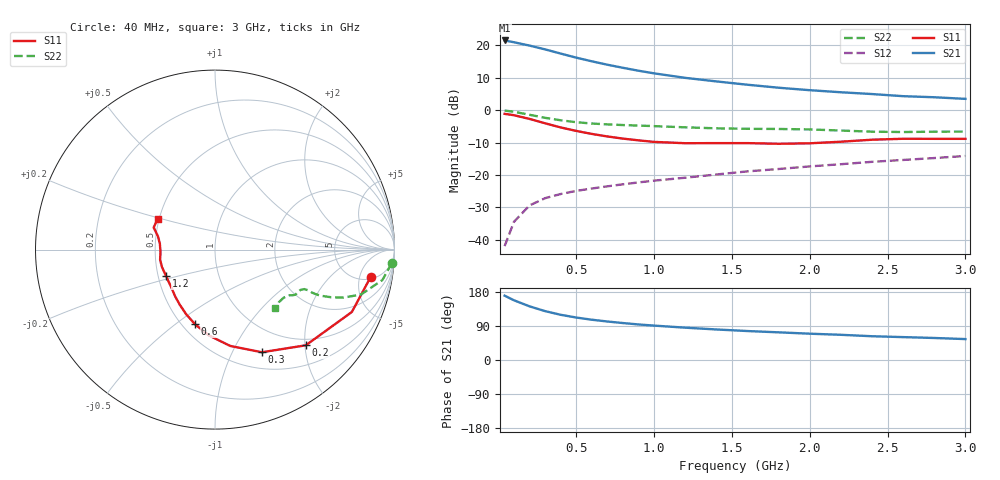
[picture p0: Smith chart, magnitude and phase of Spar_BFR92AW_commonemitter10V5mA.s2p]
! Filename:  BFR92AWG.S2P  Version:  4.0
! NXP part #: BFR92AW  Date: Jun 1994
! Bias condition: Vce=10V, Ic=5mA
#  MHz  S  MA  R  50
! Freq  S11  S21  S12  S22  !GUM [dB]
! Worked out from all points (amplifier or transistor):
!   21 points, 40 MHz to 3 GHz, reference 50 ohm
!   highest |S21| = 21.5 dB at 40 MHz (marker M1)
!   |S21| within 3 dB of that: start of sweep to 319.1 MHz
!   unconditionally stable (mu >= 1): 962.7 MHz to end of sweep
!   at 300 MHz: K = 0.48, MSG = 23.0 dB, |S12| = -27.1 dB
!   at 1 GHz: K = 1.02, MAG = 15.7 dB, |S12| = -21.7 dB
!   at 3 GHz: K = 1.14, MAG = 6.5 dB, |S12| = -14.1 dB
!   lowest NFmin = 1.60 dB at 500 MHz
!   S11 on the Smith chart (normalised r, x): 40 MHz: 5.41, -7.41; 200 MHz: 0.87, -2.02; 300 MHz: 0.69, -1.31; 600 MHz: 0.58, -0.59; 1.2 GHz: 0.55, -0.18; 3 GHz: 0.49, +0.19
40  0.88 -10.1  11.93 169.8  0.008 84.3  0.988 -4.4
100  0.838 -24.5  11.19 157.6  0.019 75.3  0.948 -10.3
200  0.735 -46.5  9.939 141.6  0.034 65.5  0.851 -17.1
300  0.629 -65.4  8.686 129.0  0.044 59.8  0.764 -20.5
400  0.543 -81.1  7.485 119.3  0.051 57.2  0.7 -22.3
500  0.48 -93.9  6.476 112.1  0.057 56.4  0.654 -23.3
600  0.431 -104.9  5.687 106.3  0.062 57.1  0.624 -23.8
700  0.394 -114.1  5.039 101.6  0.067 58.2  0.605 -23.9
800  0.365 -122.4  4.515 97.5  0.072 59.3  0.591 -23.9
900  0.343 -130.2  4.07 93.8  0.077 60.4  0.58 -23.7
1000  0.325 -137.5  3.708 90.8  0.082 61.6  0.569 -23.6
1200  0.31 -151.4  3.159 85.3  0.091 63.8  0.545 -23.8
1400  0.311 -161.9  2.785 80.6  0.102 66.0  0.526 -25.3
1600  0.311 -169.6  2.474 76.4  0.114 67.5  0.517 -27.7
1800  0.304 -177.1  2.225 73.0  0.124 69.4  0.514 -29.2
2000  0.309 173.8  2.038 69.4  0.136 70.8  0.506 -30.1
2200  0.327 166.7  1.894 66.5  0.147 72.0  0.486 -31.6
2400  0.351 162.1  1.777 62.7  0.16 72.8  0.467 -35.0
2600  0.363 160.2  1.648 60.4  0.171 73.4  0.461 -39.5
2800  0.362 156.9  1.586 58.1  0.183 74.7  0.467 -42.6
3000  0.362 151.8  1.498 55.2  0.197 75.2  0.468 -44.5
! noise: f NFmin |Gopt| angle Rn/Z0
500  1.6  0.461  15.9  0.36
1000  2.1  0.327  48  0.42
2000  3  0.174  155.6  0.26
